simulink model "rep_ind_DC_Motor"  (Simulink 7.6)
settings: Solver=ode15s  StartTime=0.0  StopTime=N  RelTol=1e-3
InitFcn:
  | N=35e-6;
  | % Paramètres mécaniques
  | J=0.01;
StopFcn:
  | close all
  | load pos_vit.mat
  | plotyy(x(1,:),x(2,:), x(1,:),x(3,:))
  | grid
  | title('Position et Vitesse d''un moteur à courant continu')
  | xlabel('temps')
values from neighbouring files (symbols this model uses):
  K = 0.0005    [parametres.m]
  R = 4    [parametres.m]    (also in Prog_callbacks.m = 1000; oscillateur_dephasage.m = 1000; Calcul_Ampl_phase_A.m = 1; circuit_RLC_parallele_.m)
libraries: fl_lib x11, nesl_utility x5

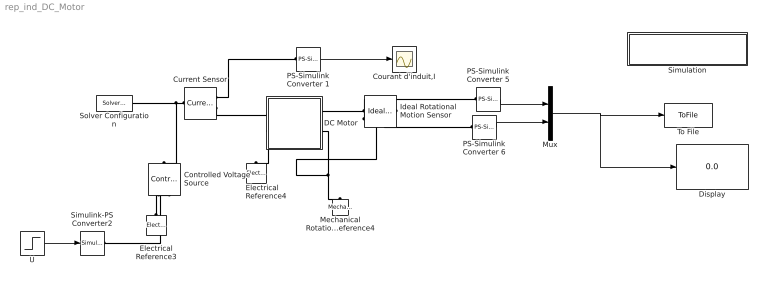
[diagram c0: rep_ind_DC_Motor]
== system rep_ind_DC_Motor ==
  Controlled Voltage Source : fl_lib/Electrical/Electrical Sources/Controlled Voltage Source  DialogController=NetworkEngine.DynNeDlgSource  SystemSampleTime=-1  i_Log=off  v_Log=off  LocalVarNames=|current|voltage|power  LocalVarDescs=|Current (A)|Voltage (V)|Power (W)  LocalVarLogging=[0 0 0]
  Courant d'induit,I : Scope
  Current Sensor : fl_lib/Electrical/Electrical Sensors/Current Sensor  DialogController=NetworkEngine.DynNeDlgSource  SystemSampleTime=-1  i1_Log=off  v1_Log=off  LocalVarNames=|i1|v1  LocalVarDescs=|i1|v1  LocalVarLogging=[0 0]
  DC Motor : Subsystem  InitFcn=|
      | Cr=0.01;   
      | R=4;L=1e-5;
      | K=0.001;
  Display : Display
  Electrical Reference3 : fl_lib/Electrical/Electrical Elements/Electrical Reference  DialogController=NetworkEngine.DynNeDlgSource  SystemSampleTime=-1  i_Log=off  LocalVarNames=|i  LocalVarDescs=|i  LocalVarLogging=[]
  Electrical Reference4 : fl_lib/Electrical/Electrical Elements/Electrical Reference  DialogController=NetworkEngine.DynNeDlgSource  SystemSampleTime=-1  i_Log=off  LocalVarNames=|i  LocalVarDescs=|i  LocalVarLogging=[]
  Ideal Rotational Motion Sensor : fl_lib/Mechanical/Mechanical Sensors/Ideal Rotational Motion Sensor  DialogController=NetworkEngine.DynNeDlgSource  SystemSampleTime=-1  offset=0 rad  w_Log=off  t_Log=off  phi_Log=off  LocalVarNames=|w|t|phi  LocalVarDescs=|w|t|phi  LocalVarLogging=[]
  Mechanical Rotational Reference4 : fl_lib/Mechanical/Rotational Elements/Mechanical Rotational Reference  DialogController=NetworkEngine.DynNeDlgSource  SystemSampleTime=-1  t_Log=off  LocalVarNames=|t  LocalVarDescs=|t  LocalVarLogging=[]
  Mux : Mux  Inputs=2
  PS-Simulink Converter 1 : nesl_utility/PS-Simulink Converter  DialogController=NetworkEngine.DynNeUtilDlgSource  SystemSampleTime=-1  PhysicalDomain=network_engine_domain  LeftPortType=input  RightPortType=output  SubClassName=ps_output  Unit=A  AffineConversion=off
  PS-Simulink Converter 5 : nesl_utility/PS-Simulink Converter  DialogController=NetworkEngine.DynNeUtilDlgSource  SystemSampleTime=-1  PhysicalDomain=network_engine_domain  LeftPortType=input  RightPortType=output  SubClassName=ps_output  Unit=rad  AffineConversion=off
  PS-Simulink Converter 6 : nesl_utility/PS-Simulink Converter  DialogController=NetworkEngine.DynNeUtilDlgSource  SystemSampleTime=-1  PhysicalDomain=network_engine_domain  LeftPortType=input  RightPortType=output  SubClassName=ps_output  Unit=rad/s  AffineConversion=off
  Simulation : Subsystem
  Simulink-PS Converter2 : nesl_utility/Simulink-PS Converter  DialogController=NetworkEngine.DynNeUtilDlgSource  SystemSampleTime=-1  PhysicalDomain=network_engine_domain  LeftPortType=input  RightPortType=output  SubClassName=ps_input  Unit=1  AffineConversion=off  InputFilterTimeConstant=.001  UdotUserProvided=0
  Solver Configuration : nesl_utility/Solver Configuration  DialogController=NetworkEngine.DynNeUtilDlgSource  SystemSampleTime=-1  PhysicalDomain=network_engine_domain  LeftPortType=input  RightPortType=generic  SubClassName=solver  Accelerate=off  Profile=off  ResidualTolerance=1e-9  MaxNonlinIter=3  MaxModeIter=2  DoFixedCost=off  UseLocalSampling=off  DoDC=off  LinearAlgebra=Sparse  LocalSolverSampleTime=.001  LocalSolverChoice=NE_BACKWARD_EULER_ADVANCER  UseLocalSolver=off
  To File : ToFile  Filename=pos_vit.mat  MatrixName=x
  U : Step  Time=0  After=12  SampleTime=0
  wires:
  U/1 -> Simulink-PS Converter2/1
  PS-Simulink Converter 5/1 -> Mux/1
  PS-Simulink Converter 6/1 -> Mux/2
  Mux/1 -> To File/1, Display/1
  PS-Simulink Converter 1/1 -> Courant d'induit,I/1
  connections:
  DC Motor/LConn2 -- Electrical Reference4/LConn1
  Ideal Rotational Motion Sensor/RConn2 -- PS-Simulink Converter 6/LConn1
  Ideal Rotational Motion Sensor/RConn3 -- PS-Simulink Converter 5/LConn1
  Electrical Reference3/LConn1 -- Controlled Voltage Source/RConn2
  Simulink-PS Converter2/RConn1 -- Controlled Voltage Source/RConn1
  DC Motor/RConn2 -- Mechanical Rotational Reference4/LConn1 -- Ideal Rotational Motion Sensor/RConn1
  DC Motor/RConn1 -- Ideal Rotational Motion Sensor/LConn1
  Current Sensor/RConn2 -- DC Motor/LConn1
  Current Sensor/LConn1 -- Controlled Voltage Source/LConn1 -- Solver Configuration/RConn1
  Current Sensor/RConn1 -- PS-Simulink Converter 1/LConn1

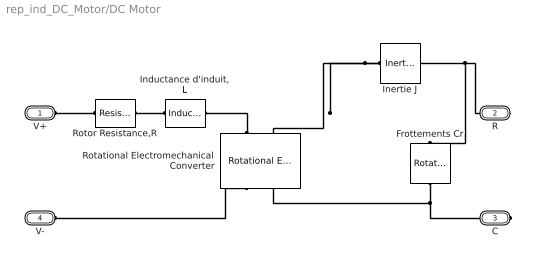
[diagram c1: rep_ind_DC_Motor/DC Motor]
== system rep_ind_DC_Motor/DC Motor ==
  Frottements Cr : fl_lib/Mechanical/Rotational Elements/Rotational Friction  DialogController=NetworkEngine.DynNeDlgSource  SystemSampleTime=-1  brkwy_trq=Cr N*m  Col_trq=Cr N*m  visc_coef=0 N*m/(rad/s)  trans_coef=10 s/rad  vel_thr=0.1 rad/s  t_Log=off  w_Log=off  LocalVarNames=|friction_torque|rel_velocity|power  LocalVarDescs=|Friction torque (N*m)|Relative velocity (rad/s)|Power (W)  LocalVarLogging=[0 0 0]
  "Inductance d'induit, L" : fl_lib/Electrical/Electrical Elements/Inductor  DialogController=NetworkEngine.DynNeDlgSource  SystemSampleTime=-1  l=L H  i0=0 A  r=0 Ohm  g=1e-09 1/Ohm  i_Log=off  v_Log=off  i_L_Log=off  LocalVarNames=|current|voltage|power  LocalVarDescs=|Inductor current (A) |Voltage across inductor (V)|Power (W)  LocalVarLogging=[0 0 0]
  Inertie J : fl_lib/Mechanical/Rotational Elements/Inertia  DialogController=NetworkEngine.DynNeDlgSource  SystemSampleTime=-1  inertia=J g*cm^2  initial_velocity=0 rad/s  t_Log=off  LocalVarNames=|torque|velocity  LocalVarDescs=|Inertia torque (N*m)|Inertia absolute velocity (rad/s)  LocalVarLogging=[0 0]
  Rotational Electromechanical Converter : fl_lib/Electrical/Electrical Elements/Rotational Electromechanical Converter  DialogController=NetworkEngine.DynNeDlgSource  SystemSampleTime=-1  K=K V/(rad/s)  i_Log=off  v_Log=off  t_Log=off  w_Log=off  LocalVarNames=|current|voltage|power|torque|speed  LocalVarDescs=|Current (A)|Voltage (V)|Power (W)|Torque (Nm)|Angular speed (rad/s)  LocalVarLogging=[0 0 0 0 0]
  Rotor Resistance,R : fl_lib/Electrical/Electrical Elements/Resistor  Tag=Factory Generic  DialogController=NetworkEngine.DynNeDlgSource  SystemSampleTime=-1  R=R Ohm  i_Log=off  v_Log=off  LocalVarNames=|current|voltage|power  LocalVarDescs=|Resistor current (A)|Voltage across resistor (V)|Power (W)  LocalVarLogging=[0 0 0]
  V+ : PMIOPort  Port=1  Side=Left
  R : PMIOPort  Port=2  Side=Right
  C : PMIOPort  Port=3  Side=Right
  V- : PMIOPort  Port=4  Side=Left
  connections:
  Frottements Cr/RConn1 -- C/RConn1 -- Rotational Electromechanical Converter/RConn2
  Inertie J/LConn1 -- Frottements Cr/LConn1 -- R/RConn1 -- Rotational Electromechanical Converter/LConn2
  "Inductance d'induit, L"/LConn1 -- Rotor Resistance,R/RConn1
  Rotor Resistance,R/LConn1 -- V+/RConn1
  V-/RConn1 -- Rotational Electromechanical Converter/RConn1
  Rotational Electromechanical Converter/LConn1 -- "Inductance d'induit, L"/RConn1

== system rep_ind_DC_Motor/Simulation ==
